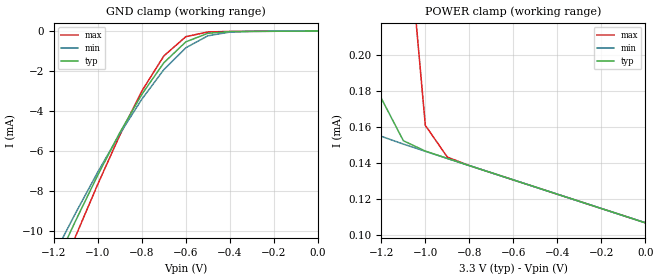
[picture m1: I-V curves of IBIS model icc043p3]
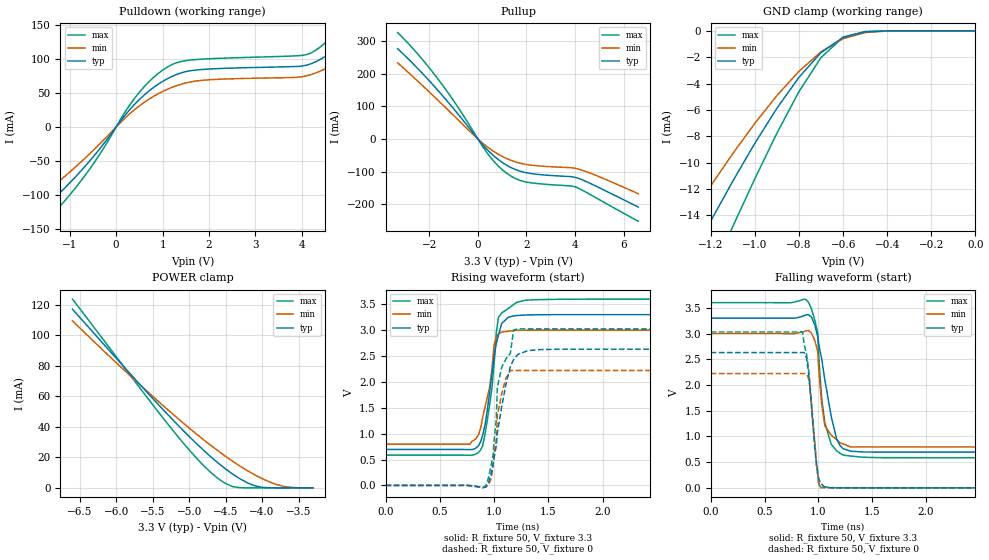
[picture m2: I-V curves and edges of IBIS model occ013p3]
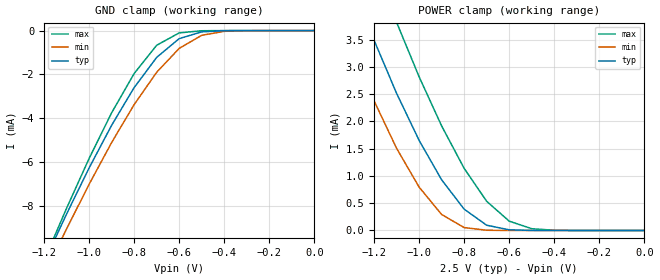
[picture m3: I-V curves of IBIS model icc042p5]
[IBIS ver]   2.1
[File name]   mpc9352.ibs
[File Rev]   2.2
[Date]   Apr 24, 2002
[Disclaimer]   This information is for modeling purposes only
|   and is not guaranteed.
[Source]   Timing Solutions Operations
[Copyright]   Copyright 2001, Motorola Incorporated,
|   all rights reserved.
| Component MPC9352 for 3.3V Application!
[Component]   MPC9352_3p3
[Manufacturer]   Motorola
[Package]
|   typ   min   max
R_pkg   0.048   0.038   0.053
L_pkg   6.045nH   5.084nH   7.950nH
C_pkg   0.813pF   0.560pF   1.157pF
[Pin] signal_name model_name R_pin   L_pin   C_pin
1   F_RANGE   icc043p3   0.04   0.35nH   0.053pF
2   F_SELC   icc043p3   0.04   0.35nH   0.053pF
3   F_SELB   icc043p3   0.04   0.35nH   0.053pF
4   F_SELA   icc043p3   0.04   0.35nH   0.053pF
5   MR/OEB   icc043p3   0.04   0.35nH   0.053pF
6   CCLK   icc043p3   0.04   0.35nH   0.053pF
8   FB_IN   icc043p3   0.04   0.35nH   0.053pF
9   PLL_ENB   icc043p3   0.04   0.35nH   0.053pF
12   QA0   occ013p3   0.04   0.35nH   0.053pF
14   QA1   occ013p3   0.04   0.35nH   0.053pF
15   QA2   occ013p3   0.04   0.35nH   0.053pF
18   QA3   occ013p3   0.04   0.35nH   0.053pF
19   QA4   occ013p3   0.04   0.35nH   0.053pF
22   QB0   occ013p3   0.04   0.35nH   0.053pF
23   QB1   occ013p3   0.04   0.35nH   0.053pF
26   QB2   occ013p3   0.04   0.35nH   0.053pF
27   QB3   occ013p3   0.04   0.35nH   0.053pF
30   QC0   occ013p3   0.04   0.35nH   0.053pF
31   QC1   occ013p3   0.04   0.35nH   0.053pF
|Component MPC9352 for 2.5V Application!
[Component]   MPC9352_2p5
[Manufacturer]   Motorola
[Package]
|   typ   min   max
R_pkg   0.048   .038   0.053
L_pkg   6.045nH   5.084nH   7.950nH
C_pkg   0.813pF   0.560pF   1.157pF
[Pin] signal_name model_name R_pin   L_pin   C_pin
1   F_RANGE   icc042p5   0.04   0.35nH   0.053pF
2   F_SELC   icc042p5   0.04   0.35nH   0.053pF
3   F_SELB   icc042p5   0.04   0.35nH   0.053pF
4   F_SELA   icc042p5   0.04   0.35nH   0.053pF
5   MR/OEB   icc042p5   0.04   0.35nH   0.053pF
6   CCLK   icc042p5   0.04   0.35nH   0.053pF
8   FB_IN   icc042p5   0.04   0.35nH   0.053pF
9   PLL_ENB   icc042p5   0.04   0.35nH   0.053pF
12   QA0   occ012p5   0.04   0.35nH   0.053pF
14   QA1   occ012p5   0.04   0.35nH   0.053pF
15   QA2   occ012p5   0.04   0.35nH   0.053pF
18   QA3   occ012p5   0.04   0.35nH   0.053pF
19   QA4   occ012p5   0.04   0.35nH   0.053pF
22   QB0   occ012p5   0.04   0.35nH   0.053pF
23   QB1   occ012p5   0.04   0.35nH   0.053pF
26   QB2   occ012p5   0.04   0.35nH   0.053pF
27   QB3   occ012p5   0.04   0.35nH   0.053pF
30   QC0   occ012p5   0.04   0.35nH   0.053pF
31   QC1   occ012p5   0.04   0.35nH   0.053pF
| Models and submodels in the file (4): icc043p3 (Input), occ013p3 (Output), icc042p5 (Input), occ012p5 (Output)
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|This model is an Input with a 25,000 ohm Pull_down at 3.3V
[Model]   icc043p3
Model_type   Input
Vref=1.5V
Vinl=0.8V
Vinh=2.0V
| Variable   typ   min   max
C_comp   5p   5p   5p
[Temperature Range]   27.00   100.00   -45.00
[Power Clamp Reference]   3.30V   3.00V   3.60V
[Gnd Clamp Reference]   0.000V   0.000V   0.000V
[Voltage Range]   3.30V   3.00V   3.60V
[Pulldown Reference]   0.000V   0.000V   0.000V
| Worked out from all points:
|   GND clamp passes 1 mA (typ) near -0.64 V on its own axis
|   POWER clamp passes 1 mA (typ) near -1.44 V on its own axis
[GND_clamp]
| voltage   I(typ)   I(min)   I(max)
-3.3V     -65.45mA   -61.69mA   -70.25mA
-1.2V     -11.83mA   -11.21mA   -12.91mA
-1.1V     -9.467mA   -9.084mA   -10.24mA
-1V       -7.201mA   -7.048mA   -7.655mA
-900mV    -5.077mA   -5.139mA   -5.207mA
-800mV    -3.163mA   -3.405mA   -2.998mA
-700mV    -1.585mA   -1.928mA   -1.242mA
-600mV    -537uA     -834.6uA   -278.5uA
-500mV    -111.2uA   -235.5uA   -44.5uA
-400mV    -25.07uA   -49.72uA   -17.01uA
1.97fV    -61.68pA   -9.69nA    -3.014pA
[POWER_clamp]
| voltage   I(typ)  I(min)  I(max)
-3.3V     27.21mA    21.56mA    34.07mA
-1.5V     1.4mA      337.1uA    3.859mA
-1.4V     717.9uA    194.4uA    2.632mA
-1.3V     311.6uA    162.1uA    1.579mA
-1.2V     175.9uA    154.8uA    767.8uA
-1.1V     152.4uA    150.5uA    297.2uA
-1V       146.6uA    146.5uA    160.9uA
-900mV    142.6uA    142.6uA    143.3uA
-800mV    138.6uA    138.6uA    138.6uA
1.97fV    106.9uA    106.9uA    106.9uA
|  Output Buffer at 3.3V Application
[Model]   occ013p3
Model_type   Output
Enable   Active-Low
Polarity   Non-Inverting
Vref=1.5
Cref=1pf
Rref=50
| Variable   typ   min   max
C_comp   5p   5p   5p
[Temperature Range]   27.00   100.00   -45.00
[Voltage Range]   3.30V   3.00V   3.60V
[Pulldown Reference]   0.000V   0.000V   0.000V
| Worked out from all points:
|   slope of the pulldown table from 0 to 0.495 V, typ, clamps not added: 12.4 ohm
|   slope of the pullup table from 0 to 0.495 V, typ, clamps not added: 12.1 ohm
|   GND clamp passes 1 mA (typ) near -0.64 V on its own axis
|   POWER clamp passes 1 mA (typ) near -4.06 V on its own axis
|   rising waveform, R_fixture 50, V_fixture 3.3: 20-80 % time 105ps typ, 105ps min, 91.8ps max; typ from 0.695 V to 3.3 V
|   falling waveform, R_fixture 50, V_fixture 3.3: 20-80 % time 133ps typ, 61.6ps min, 76.5ps max; typ from 3.3 V to 0.695 V
|   rising waveform, R_fixture 50, V_fixture 0: 20-80 % time 127ps typ, 77.6ps min, 112ps max; typ from 0 V to 2.63 V
|   falling waveform, R_fixture 50, V_fixture 0: 20-80 % time 63.4ps typ, 54ps min, 76.3ps max; typ from 2.63 V to 0 V
[Pulldown]
|Voltage   I(typ)   I(min)   I(max)
-3.3V     -209.8mA   -184.1mA   -233.1mA
-2.5V     -171.4mA   -145.7mA   -196.3mA
-2V       -144.6mA   -120.9mA   -169.9mA
-1.6V     -121.3mA   -100.1mA   -144.4mA
-600mV    -52.28mA   -41.26mA   -64.61mA
500mV     40.26mA    30.94mA    50.94mA
1.2V      74.05mA    58.02mA    91.38mA
4.1V      90.56mA    75mA       106.1mA
4.8V      118.5mA    95.76mA    145.2mA
5.2V      146.1mA    114.5mA    186.5mA
5.7V      200mA      148.6mA    270.9mA
6.6V      419.9mA    278.5mA    628.6mA
[Pullup]
|Voltage   I(typ)   I(min)   I(max)
-3.3V     276.2mA    233mA      325.6mA
-2.5V     217.6mA    178.8mA    262.3mA
-1.7V     153.4mA    122.6mA    189.2mA
-800mV    74.59mA    57.3mA     95.02mA
300mV     -26.06mA   -19.2mA    -34.48mA
700mV     -54.72mA   -40.53mA   -71.91mA
1.1V      -76.73mA   -57.15mA   -100.1mA
1.5V      -92.4mA    -69.23mA   -119.7mA
1.9V      -102.1mA   -76.99mA   -130.5mA
4V        -117.6mA   -89.99mA   -146.7mA
4.8V      -142.5mA   -110mA     -177.7mA
6.6V      -208.6mA   -167.9mA   -252.3mA
[GND_clamp]
|Voltage   I(typ)   I(min)   I(max)
-3.3V     -85.27mA   -74.38mA   -97.87mA
-1.4V     -20.76mA   -16.98mA   -26.15mA
-1.3V     -17.56mA   -14.32mA   -22.34mA
-1.2V     -14.43mA   -11.76mA   -18.57mA
-1.1V     -11.4mA    -9.311mA   -14.84mA
-900mV    -5.871mA   -4.914mA   -7.763mA
-800mV    -3.524mA   -3.07mA    -4.613mA
-700mV    -1.653mA   -1.587mA   -2.027mA
-600mV    -494uA     -597.7uA   -480.9uA
-500mV    -78.44uA   -130.1uA   -51.01uA
-400mV    -7.209uA   -15.25uA   -2.718uA
1.97fV    -33.27pA   -701.5pA   -3.87pA
[POWER_clamp]
|Voltage   I(typ)   I(min)   I(max)
-6.6V     117mA      109.4mA    123.6mA
-5.8V     74.29mA    73.06mA    73.28mA
-5.2V     43.37mA    47.3mA     36.28mA
-4.9V     29.01mA    35.26mA    19.52mA
-4.6V     16.15mA    24.09mA    5.976mA
-4.5V     12.36mA    20.62mA    2.814mA
-4.4V     8.904mA    17.3mA     800.8uA
-4.2V     3.283mA    11.23mA    5.412uA
-4.1V     1.379mA    8.513mA    174.8nA
-3.9V     43.18uA    3.908mA    72.88pA
-3.7V     227.2nA    935.3uA    4.59pA
-3.3V     48.11pA    322.6nA    3.568pA
[Ramp]
dV/dt_r   1.56/105p   1.29/169p   1.81/69.3p
dV/dt_f   1.56/127.4p   1.3/192.1p   1.81/88.1p
R_load = 50
[Rising Waveform]
R_fixture = 50
V_fixture = 3.3
V_fixture_min = 3.0
V_fixture_max = 3.6
|Time (ns) Voltage(typ)  Voltage(min)  Voltage(max)
0s        695mV      795.2mV    585.3mV
776ps     691.2mV    795.2mV    581.3mV
858ps     771.9mV    985.6mV    638mV
895ps     972.8mV    1.315V     766.3mV
958ps     1.778V     1.889V     1.542V
1ns       2.487V     2.722V     2.333V
1.04ns    2.904V     2.926V     3.247V
1.07ns    3.129V     2.965V     3.333V
1.21ns    3.283V     2.998V     3.539V
5ns       3.3V       3V         3.6V
[Falling Waveform]
R_fixture = 50
V_fixture = 3.3
V_fixture_min = 3.0
V_fixture_max = 3.6
|Time (ns) Voltage(typ)  Voltage(min)  Voltage(max)
0s        3.3V       3V         3.6V
908ps     3.368V     3.061V     3.608V
994ps     2.939V     2.654V     3.01V
1.01ns    2.718V     2.137V     2.349V
1.03ns    2.52V      1.654V     1.761V
1.06ns    2.104V     1.21V      1.263V
1.12ns    1.384V     1.023V     846.3mV
1.17ns    950.1mV    937.9mV    721mV
1.23ns    761.7mV    854.5mV    637.3mV
5ns       695mV      795.3mV    585.3mV
[Rising Waveform]
R_fixture = 50
V_fixture = 0
V_fixture_min = 0
V_fixture_max = 0
|Time (ns) Voltage(typ)  Voltage(min)  Voltage(max)
0s        286.8pV    9.073nV    24.07pV
924ps     -30.9mV    -32.03mV   -10.33mV
991ps     416.9mV    374.4mV    591mV
1.02ns    757mV      893.3mV    1.26V
1.03ns    1.015V     1.343V     1.899V
1.11ns    1.961V     2.075V     2.446V
1.15ns    2.296V     2.221V     2.553V
1.18ns    2.432V     2.221V     3.004V
1.43ns    2.625V     2.221V     3.025V
5ns       2.632V     2.221V     3.025V
[Falling Waveform]
R_fixture = 50
V_fixture = 0
V_fixture_min = 0
V_fixture_max = 0
|Time (ns) Voltage(typ)  Voltage(min)  Voltage(max)
0s        2.63V      2.222V     3.03V
853ps     2.63V      2.222V     3.03V
890ps     2.524V     2.217V     2.597V
919ps     2.025V     1.996V     2.099V
966ps     783.7mV    921.9mV    881.6mV
982ps     456.5mV    459.8mV    514.4mV
1ns       209.4mV    107mV      137.6mV
1.02ns    95.09mV    4.92mV     24.83mV
1.1ns     3.325mV    2.05mV     9.039mV
5ns       -11.9uV    304.1nV    11.65uV
|This model is an Input with a 25,000 ohm Pull_down at 2.5V
[Model]   icc042p5
Model_type   Input
Vmeas=1.25V
Vinl=0.7V
Vinh=1.7V
| Variable   typ   min   max
C_comp   5p   5p   5p
[Temperature Range]   27.00   100.00   -45.00
[Power Clamp Reference]   2.50V   2.25V   2.75V
[Gnd Clamp Reference]   0.000V   0.000V   0.000V
[Voltage Range]   2.50V   2.25V   2.75V
[Pulldown Reference]   0.000V   0.000V   0.000V
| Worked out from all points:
|   GND clamp passes 1 mA (typ) near -0.67 V on its own axis
|   POWER clamp passes 1 mA (typ) near -0.91 V on its own axis
[GND_clamp]
| voltage   I(typ)   I(min)   I(max)
-2.5V     -42.32mA   -41.95mA   -44.12mA
-1.2V     -10.57mA   -11.17mA   -10.49mA
-1.1V     -8.363mA   -9.042mA   -8.101mA
-1V       -6.263mA   -7.009mA   -5.833mA
-900mV    -4.318mA   -5.104mA   -3.748mA
-800mV    -2.598mA   -3.374mA   -1.958mA
-700mV    -1.223mA   -1.901mA   -669.1uA
-600mV    -367.4uA   -811uA     -105.4uA
-500mV    -58.52uA   -215.8uA   -8.126uA
-400mV    -5.383uA   -33.88uA   -283nA
1.08fV    -5.997pA   -3.129nA   -2.5pA
[POWER_clamp]
| voltage   I(typ)  I(min)  I(max)
-2.5V     20.92mA    19.68mA    22.84mA
-1.4V     5.706mA    4.479mA    7.266mA
-1.3V     4.561mA    3.379mA    6.054mA
-1.2V     3.493mA    2.381mA    4.903mA
-1.1V     2.518mA    1.509mA    3.822mA
-1V       1.655mA    796.6uA    2.822mA
-900mV    930.3uA    293.6uA    1.919mA
-800mV    391.2uA    53.28uA    1.14mA
-700mV    96.35uA    4.13uA     535.5uA
-600mV    12.19uA    177.5nA    171.1uA
-500mV    1.038uA    4.826nA    32.15uA
1.08fV    126pA      102.5pA    3.439nA
